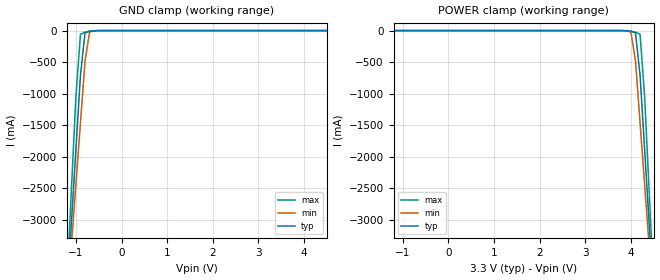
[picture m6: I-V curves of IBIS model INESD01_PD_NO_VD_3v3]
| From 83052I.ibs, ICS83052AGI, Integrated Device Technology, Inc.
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[Model] INESD01_PD_NO_VD_3v3
Model_type   Input
Polarity   Non-Inverting
Vinl = 0.80V
Vinh = 2.0V
|   typ   min   max
C_comp   2pF   1.5pF   2.5pF
|   typ   min   max
[Voltage range]  3.3V   3.135V   3.465V
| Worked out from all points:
|   GND clamp passes 1 mA (typ) near -0.53 V on its own axis
[GND_clamp]
|Voltage I(typ)   I(min)   I(max)
-3.3V     -29.06A    -25.07A    -35.75A
-1.2V     -4.247A    -4.404A    -4.063A
-1.1V     -3.067A    -3.422A    -2.554A
-1V       -1.887A    -2.441A    -1.045A
-900mV    -707.9mA   -1.461A    -58.38mA
-800mV    -36.14mA   -481.4mA   -25.07mA
-700mV    -7.313mA   -24.33mA   -13.7mA
-600mV    -2.207mA   -1.763mA   -5.095mA
6.6V      128.6uA    160.8uA    121.8uA
[POWER_clamp]
|Voltage   I(typ)   I(min)   I(max)
-3.3V     128.6uA    160.8uA    121.8uA
3.9V      -2.207mA   -1.763mA   -5.095mA
4V        -7.314mA   -24.33mA   -13.7mA
4.1V      -36.14mA   -481.4mA   -25.07mA
4.2V      -707.9mA   -1.461A    -58.38mA
4.3V      -1.887A    -2.441A    -1.045A
4.4V      -3.067A    -3.422A    -2.554A
4.5V      -4.247A    -4.404A    -4.063A
6.6V      -29.06A    -25.07A    -35.75A
